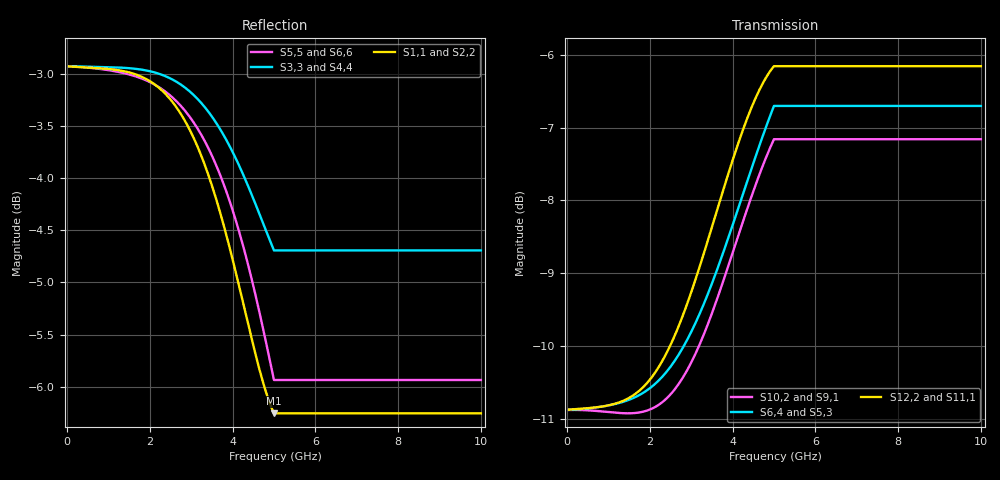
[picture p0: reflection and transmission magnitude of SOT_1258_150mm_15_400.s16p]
! Created Sun Apr 17 16:15:13 2016
! 16 Port Network Data from SP1.SP block
! freq  magS1_1  angS1_1  magS1_2  angS1_2  magS1_3  angS1_3  magS1_4  angS1_4
!  magS1_5  angS1_5  magS1_6  angS1_6  magS1_7  angS1_7  magS1_8  angS1_8
!  magS1_9  angS1_9  magS1_10  angS1_10  magS1_11  angS1_11  magS1_12  angS1_12
!  magS1_13  angS1_13  magS1_14  angS1_14  magS1_15  angS1_15  magS1_16  angS1_16
!  magS2_1  angS2_1  magS2_2  angS2_2  magS2_3  angS2_3  magS2_4  angS2_4
!  magS2_5  angS2_5  magS2_6  angS2_6  magS2_7  angS2_7  magS2_8  angS2_8
!  magS2_9  angS2_9  magS2_10  angS2_10  magS2_11  angS2_11  magS2_12  angS2_12
!  magS2_13  angS2_13  magS2_14  angS2_14  magS2_15  angS2_15  magS2_16  angS2_16
!  magS3_1  angS3_1  magS3_2  angS3_2  magS3_3  angS3_3  magS3_4  angS3_4
!  magS3_5  angS3_5  magS3_6  angS3_6  magS3_7  angS3_7  magS3_8  angS3_8
!  magS3_9  angS3_9  magS3_10  angS3_10  magS3_11  angS3_11  magS3_12  angS3_12
!  magS3_13  angS3_13  magS3_14  angS3_14  magS3_15  angS3_15  magS3_16  angS3_16
!  magS4_1  angS4_1  magS4_2  angS4_2  magS4_3  angS4_3  magS4_4  angS4_4
!  magS4_5  angS4_5  magS4_6  angS4_6  magS4_7  angS4_7  magS4_8  angS4_8
!  magS4_9  angS4_9  magS4_10  angS4_10  magS4_11  angS4_11  magS4_12  angS4_12
!  magS4_13  angS4_13  magS4_14  angS4_14  magS4_15  angS4_15  magS4_16  angS4_16
!  magS5_1  angS5_1  magS5_2  angS5_2  magS5_3  angS5_3  magS5_4  angS5_4
!  magS5_5  angS5_5  magS5_6  angS5_6  magS5_7  angS5_7  magS5_8  angS5_8
!  magS5_9  angS5_9  magS5_10  angS5_10  magS5_11  angS5_11  magS5_12  angS5_12
!  magS5_13  angS5_13  magS5_14  angS5_14  magS5_15  angS5_15  magS5_16  angS5_16
!  magS6_1  angS6_1  magS6_2  angS6_2  magS6_3  angS6_3  magS6_4  angS6_4
!  magS6_5  angS6_5  magS6_6  angS6_6  magS6_7  angS6_7  magS6_8  angS6_8
!  magS6_9  angS6_9  magS6_10  angS6_10  magS6_11  angS6_11  magS6_12  angS6_12
!  magS6_13  angS6_13  magS6_14  angS6_14  magS6_15  angS6_15  magS6_16  angS6_16
!  magS7_1  angS7_1  magS7_2  angS7_2  magS7_3  angS7_3  magS7_4  angS7_4
!  magS7_5  angS7_5  magS7_6  angS7_6  magS7_7  angS7_7  magS7_8  angS7_8
!  magS7_9  angS7_9  magS7_10  angS7_10  magS7_11  angS7_11  magS7_12  angS7_12
!  magS7_13  angS7_13  magS7_14  angS7_14  magS7_15  angS7_15  magS7_16  angS7_16
!  magS8_1  angS8_1  magS8_2  angS8_2  magS8_3  angS8_3  magS8_4  angS8_4
!  magS8_5  angS8_5  magS8_6  angS8_6  magS8_7  angS8_7  magS8_8  angS8_8
!  magS8_9  angS8_9  magS8_10  angS8_10  magS8_11  angS8_11  magS8_12  angS8_12
!  magS8_13  angS8_13  magS8_14  angS8_14  magS8_15  angS8_15  magS8_16  angS8_16
!  magS9_1  angS9_1  magS9_2  angS9_2  magS9_3  angS9_3  magS9_4  angS9_4
!  magS9_5  angS9_5  magS9_6  angS9_6  magS9_7  angS9_7  magS9_8  angS9_8
!  magS9_9  angS9_9  magS9_10  angS9_10  magS9_11  angS9_11  magS9_12  angS9_12
!  magS9_13  angS9_13  magS9_14  angS9_14  magS9_15  angS9_15  magS9_16  angS9_16
!  magS10_1  angS10_1  magS10_2  angS10_2  magS10_3  angS10_3  magS10_4  angS10_4
!  magS10_5  angS10_5  magS10_6  angS10_6  magS10_7  angS10_7  magS10_8  angS10_8
!  magS10_9  angS10_9  magS10_10  angS10_10  magS10_11  angS10_11  magS10_12  angS10_12
!  magS10_13  angS10_13  magS10_14  angS10_14  magS10_15  angS10_15  magS10_16  angS10_16
!  magS11_1  angS11_1  magS11_2  angS11_2  magS11_3  angS11_3  magS11_4  angS11_4
!  magS11_5  angS11_5  magS11_6  angS11_6  magS11_7  angS11_7  magS11_8  angS11_8
!  magS11_9  angS11_9  magS11_10  angS11_10  magS11_11  angS11_11  magS11_12  angS11_12
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# ghz S ma R 50
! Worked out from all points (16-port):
!   200 points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, 50 MHz to 10 GHz, reference 50 ohm
!   strongest paths, dB at 50 MHz, 2.55 GHz, 5.05 GHz, 7.55 GHz, 10 GHz:
!     S12,2: -10.9, -9.9, -6.2, -6.2, -6.2
!     S11,1: -10.9, -9.9, -6.2, -6.2, -6.2
!     S6,4: -10.9, -10.2, -6.7, -6.7, -6.7
!     S5,3: -10.9, -10.2, -6.8, -6.8, -6.8
!     S10,2: -10.9, -10.6, -7.2, -7.2, -7.2
!     S9,1: -10.9, -10.6, -7.2, -7.2, -7.2
!   lowest |S11| = -6.3 dB at 5 GHz (marker M1), VSWR 2.90, Z = 17.4 + j4.29 ohm
!   |S11| at or under -10 dB: nowhere
